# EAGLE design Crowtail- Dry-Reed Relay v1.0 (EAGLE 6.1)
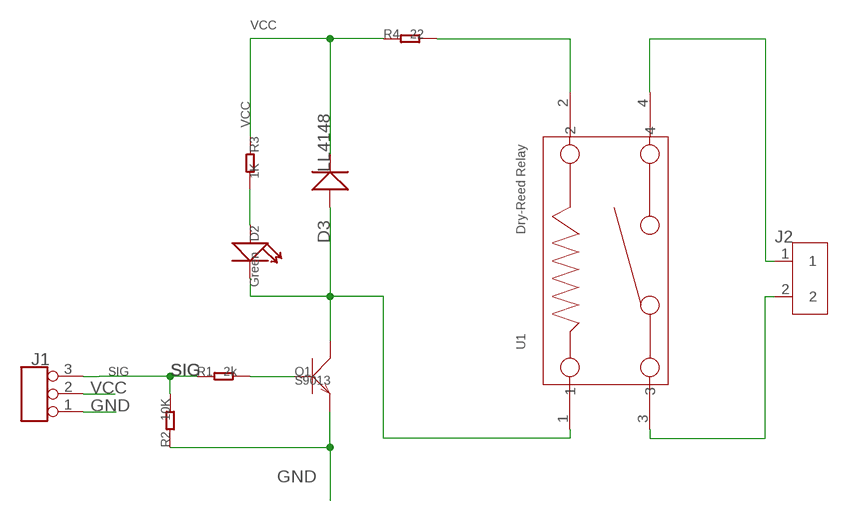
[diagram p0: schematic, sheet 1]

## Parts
D2  Green  LED'0603'  [LED-0603]
D3  LL4148  D'1N4148-SMD'  [DO-35-SMD]
J1  TINKER_3P_DIP  [3P_2.0_DIP]
J2  SCREW-TERMINAL-2P'5.08'  [2P-5.08]
Q1  S9013  TRANSISTOR-NPN-SOT23  [SOT23]
R1  2k  R-0603  [R0603]
R2  10K  R-0603  [R0603]
R3  1K  R-0603  [R0603]
R4  22  R-0603  [R0603]
U1  Dry-Reed Relay  RELAY-BR'BR-500R-H-5VDC'  [4P-25.2X8X9H]

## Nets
GND: J1.1 Q1.2(E) R2.1
N$1: Q1.1(B) R1.2
N$2: D2.+ R3.2
N$3: D2.- D3.A(+) Q1.3(C) U1.1
N$5: J2.1 U1.4
N$6: J2.2 U1.3
N$12: R4.2 U1.2
SIG: J1.3 R1.1 R2.2
VCC: D3.C(-) J1.2 R3.1 R4.1

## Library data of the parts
D2 = Discrete:LED*
D3 = Discrete:D*
J1 = Connector:TINKER_3P_DIP
J2 = Connector:SCREW-TERMINAL-2P
Q1 = Discrete:TRANSISTOR-NPN*: NPN audion
R1-R4 = Discrete:R*
U1 = template:RELAY-BR: • Small size, light weight and low cost • Application: Mainly use in Cordless Phone, Answering Machine and Security Alarm System etc.… • UL File No.E147052

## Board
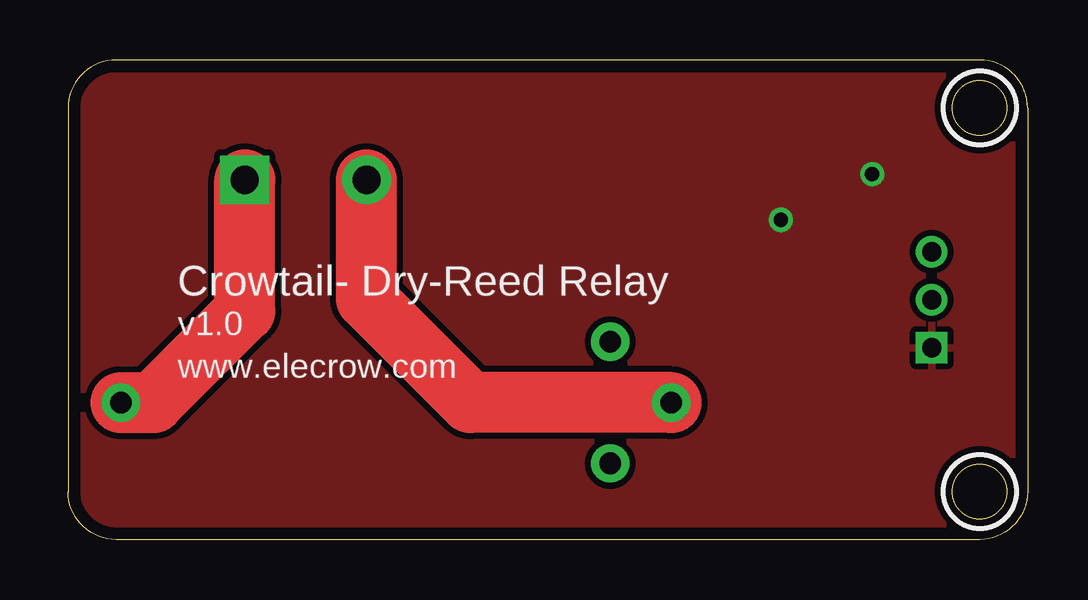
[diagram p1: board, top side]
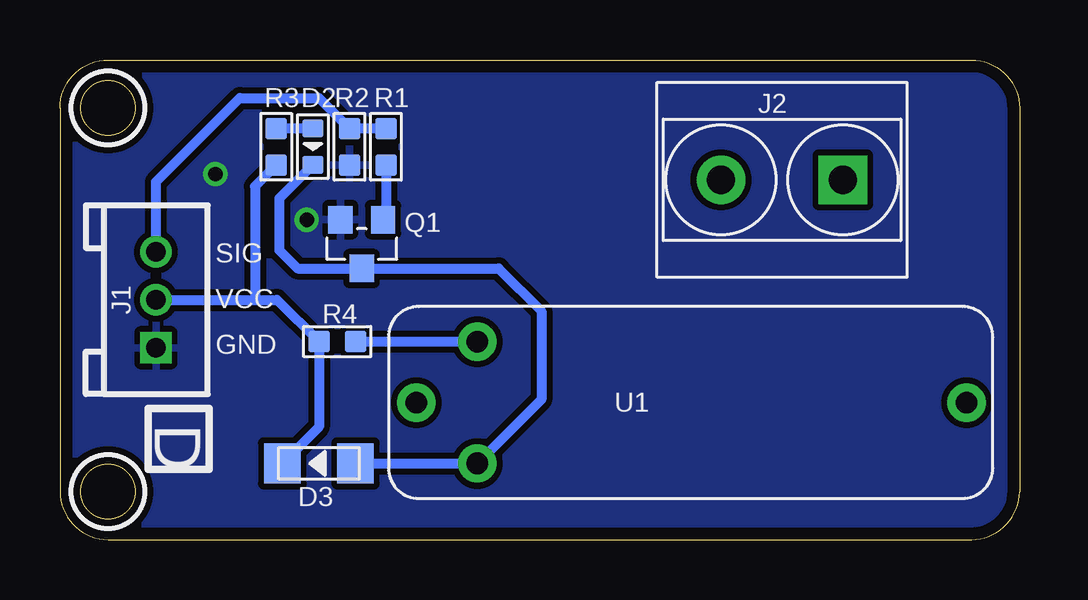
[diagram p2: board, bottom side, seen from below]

Size 40 x 20 mm. Coordinates in mm from the lower left corner, seen from the top.
Outline: 40,18 40,2 arc-90 38,0 2,0 arc-90 0,2 0,18 arc-90 2,20 38,20 arc-90 40,18
Outline: circle at 38,18 radius 1.14
Outline: circle at 38,18 radius 1.14
Outline: circle at 38,2 radius 1.14
Copper layers (1*16): Top 0.035mm / dielectric 1.5mm / Bottom 0.035mm
Design rules "default *": minimum track width 10mil, minimum drill 24mil, track to track 8mil, track to pad 8mil, pad to pad 8mil, via to via 8mil, smd to smd 8mil, copper to edge 20mil, drill to drill 8mil, minimum pad ring 10mil, minimum via ring 8mil, stop-mask expansion 4mil, vias tented up to drill 100mil, thermal gap 10mil
tRestrict: area 36.5,16.5 to 39.5,19.5; area 36.5,0.5 to 39.5,3.5
bRestrict: area 36.5,16.5 to 39.5,19.5; area 36.5,0.5 to 39.5,3.5

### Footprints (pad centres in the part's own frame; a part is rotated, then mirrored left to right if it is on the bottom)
LED-0603 = smd 0.762 x 0.889: + -0.762,0; - 0.762,0
DO-35-SMD = smd 1.524 x 1.676: A -1.524,0; C 1.524,0
3P_2.0_DIP = drill 0.8 pad 1.27 square: 1 -2,0 | drill 0.8 pad 1.27: 2 0,0; 3 2,0
2P-5.08 = drill 1.168 pad 2.032 square: 1 0,2.54 | drill 1.168 pad 2.032: 2 0,-2.54
SOT23 = smd 1.016 x 1.143: 1 -0.889,-1.016; 2 0.889,-1.016; 3 0,1.016
R0603 = smd 0.889 x 0.889: 1 -0.762,0; 2 0.762,0
4P-25.2X8X9H = drill 0.9 pad 1.6: 1 -8.89,-2.54; 2 -8.89,2.54; 3 -11.43,0; 4 11.51,0

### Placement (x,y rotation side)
D2  29.46,16.38 270 bottom
D3  29.2,3.17 180 bottom
J1  36,10 90 bottom
J2  9.9,15 270 bottom
Q1  27.42,12.32 180 bottom
R1  26.41,16.38 270 bottom
R2  27.93,16.38 90 bottom
R3  30.98,16.38 90 bottom
R4  28.44,8.26 0 bottom
U1  13.71,5.71 0 bottom

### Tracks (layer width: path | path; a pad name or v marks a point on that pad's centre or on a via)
GND  (via drill 0.6)
  other vias: 33.52,15.24 29.71,13.34
  pour Bottom (isolate 0.254): 40.76,20.83 -0.89,20.83 -0.89,-0.64 40.76,-0.64
  pour Top (isolate 0.254): 40.63,20.7 -0.77,20.7 -0.77,-0.51 40.63,-0.51
N$1
  Bottom 0.406: R1.2 26.41,13.59 26.54,13.46 Q1.1
N$2
  Bottom 0.406: D2.+ R3.2
N$3
  Bottom 0.406: D3.A U1.1 19.93,5.84 19.93,9.53 21.72,11.31 Q1.3 30.09,11.3 30.86,12.06 30.86,14.22 D2.-
N$5
  Top 2.54: U1.4 3.55,5.71 7.36,9.53 J2.1
N$6
  Top 2.54: U1.3 16.76,5.71 12.44,10.03 J2.2
N$12
  Bottom 0.406: R4.2 U1.2
SIG
  Bottom 0.406: R1.1 R2.2 29.2,18.41 32.51,18.41 36,14.92 J1.3
VCC
  Bottom 0.406: J1.2 31.87,10 | 31.87,10 30.95,10 R4.1 29.2,4.7 D3.C | R3.1 31.87,14.73 31.87,10

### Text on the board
tPlace: Crowtail- Dry-Reed Relay | v1.0 | www.elecrow.com
bPlace: D
bNames: SIG | VCC | GND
